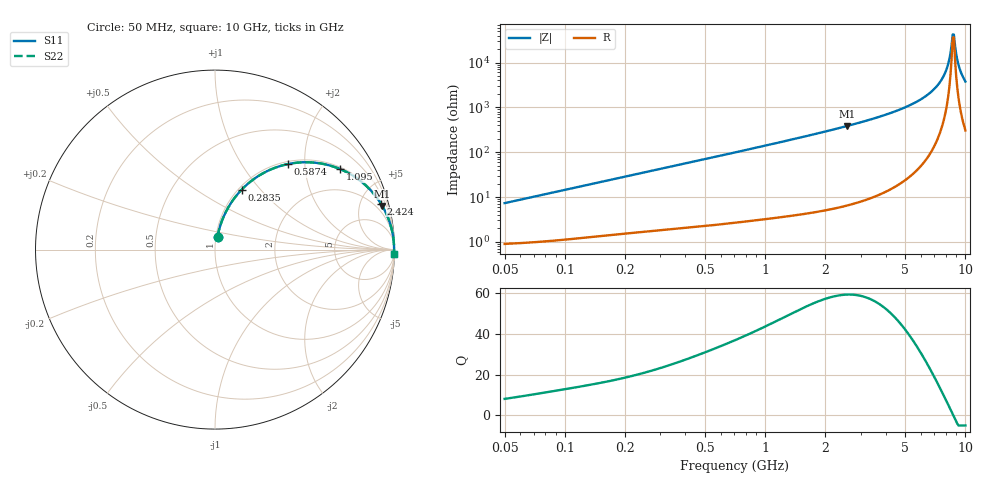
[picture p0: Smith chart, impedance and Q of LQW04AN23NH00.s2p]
!Murata Part Number: LQW04AN23NH00
!These Parameters are Measured in Series Mode Connection
!  o--[Z]--o
!Port1  Port2
!  o-------o
!Freq. Start=50[MHz] Stop=10[GHz], 401[Steps]
# Hz S RI R 50
!Freq.(Hz)	S 11(Real)	S 11(Imag)	S 21(Real)	S 21(Imag)	S 12(Real)	S 12(Imag)	S 22(Real)	S 22(Imag)
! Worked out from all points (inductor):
!   401 points, 50 MHz to 10 GHz, reference 50 ohm
!   read as one part in series: L = 23.1 nH near 51.34 MHz
!   highest Q = 59.4 at 2.556 GHz (marker M1), where L = 23.8 nH
!   self-resonance near 8.644 GHz
!   S11 on the Smith chart (normalised r, x): 50 MHz: 1.02, +0.15; 283.5 MHz: 1.04, +0.80; 587.4 MHz: 1.05, +1.64; 1.095 GHz: 1.07, +3.07; 2.424 GHz: 1.12, +7.19; 10 GHz: 7, -75
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5e7  0.014 0.071  0.986 -0.071  0.986 -0.071  0.014 0.071
1.214486e8  0.0405 0.1651  0.9595 -0.1651  0.9595 -0.1651  0.0405 0.1651
2.835028e8  0.1485 0.334  0.8515 -0.334  0.8515 -0.334  0.1485 0.334
2.949953e8  0.1578 0.3435  0.8422 -0.3435  0.8422 -0.3435  0.1578 0.3435
5.874203e8  0.4056 0.4764  0.5944 -0.4764  0.5944 -0.4764  0.4056 0.4764
7.071068e8  0.4943 0.4866  0.5057 -0.4866  0.5057 -0.4866  0.4943 0.4866
1.094763e9  0.6985 0.4481  0.3015 -0.4481  0.3015 -0.4481  0.6985 0.4481
1.717543e9  0.8533 0.3448  0.1467 -0.3448  0.1467 -0.3448  0.8533 0.3448
2.423676e9  0.9245 0.2559  0.0755 -0.2559  0.0755 -0.2559  0.9245 0.2559
2.555552e9  0.9324 0.2427  0.0676 -0.2427  0.0676 -0.2427  0.9324 0.2427
4.171863e9  0.9792 0.1334  0.0208 -0.1334  0.0208 -0.1334  0.9792 0.1334
5.733131e9  0.9924 0.0735  0.00764 -0.0735  0.00764 -0.0735  0.9924 0.0735
7.086521e9  0.9966 0.0362  0.00336 -0.0362  0.00336 -0.0362  0.9966 0.0362
7.571744e9  0.9974 0.0247  0.00264 -0.0247  0.00264 -0.0247  0.9974 0.0247
7.983737e9  0.9977 0.0154  0.00226 -0.0154  0.00226 -0.0154  0.9977 0.0154
8.198065e9  0.9979 0.0107  0.00213 -0.0107  0.00213 -0.0107  0.9979 0.0107
8.530394e9  0.998 0.00359  0.00204 -0.00359  0.00204 -0.00359  0.998 0.00359
8.644138e9  0.998 0.0012  0.00203 -0.0012  0.00203 -0.0012  0.998 0.0012
8.876195e9  0.9979 -0.00362  0.00206 0.00362  0.00206 0.00362  0.9979 -0.00362
9.236013e9  0.9978 -0.011  0.00219 0.011  0.00219 0.011  0.9978 -0.011
9.48396e9  0.9977 -0.016  0.00234 0.016  0.00234 0.016  0.9977 -0.016
1e10  0.9972 -0.0263  0.00284 0.0263  0.00284 0.0263  0.9972 -0.0263
